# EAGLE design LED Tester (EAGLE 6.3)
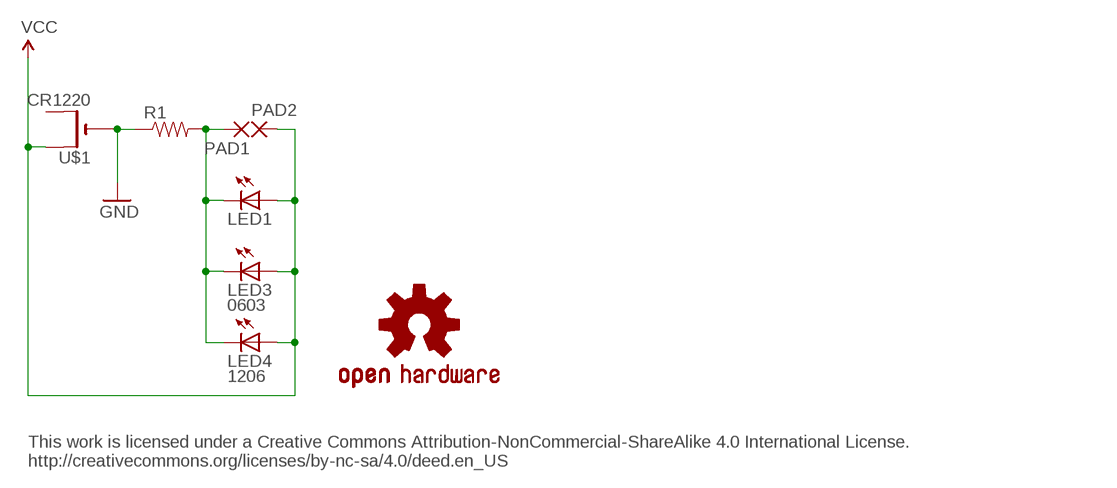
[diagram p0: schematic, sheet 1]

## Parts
LED1  LED3MM  [LED3MM]
LED3  0603  LED0603  [LED-0603]
LED4  1206  LED1206  [LED-1206]
LOGO1  OSHW-LOGOS  [OSHW-LOGO-S]
PAD1  SMD5  [SMD2,54-5,08]
PAD2  SMD5  [SMD2,54-5,08]
R1  RESISTOR0805-RES  [0805]
U$1  CR1220  CR1220THM  [CR1220-THM]

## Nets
GND: R1.1 U$1.-
N$1: LED1.K(C) LED3.C LED4.C PAD1.1(P) R1.2
VCC: LED1.A LED3.A LED4.A PAD2.1(P) U$1.+1(+)
Unconnected: U$1.+2(+1)

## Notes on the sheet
- This work is licensed under a Creative Commons Attribution-NonCommercial-ShareAlike 4.0 International License.
  http://creativecommons.org/licenses/by-nc-sa/4.0/deed.en_US

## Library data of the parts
LED1 LED3 LED4 = SparkFun-LED:LED: LEDs
LOGO1 = SparkFun-Aesthetics:OSHW-LOGO: Open Source Hardware Logo This logo indicates the piece of hardware it is found on incorporates a OSHW license and/or adheres to the definition of open source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
PAD1 PAD2 = wirepad:SMD5: SMD PAD
R1 = SparkFun-Resistors:RESISTOR: Resistor
U$1 = adafruit:CR1220: CR1216/CR1220/CR1225 12mm 3V lithium coin cell Great for battery packup. Both SMT and THM holders. Note the THM package has the ground pads on both sides of the PCB so that the masks are the same - this reduces the cost

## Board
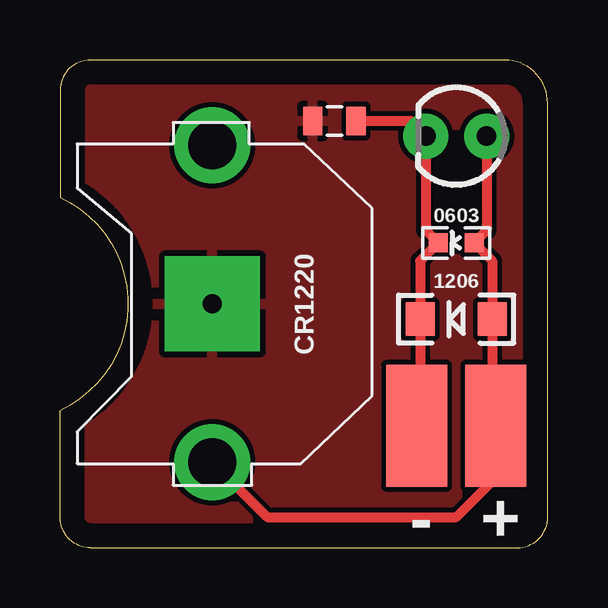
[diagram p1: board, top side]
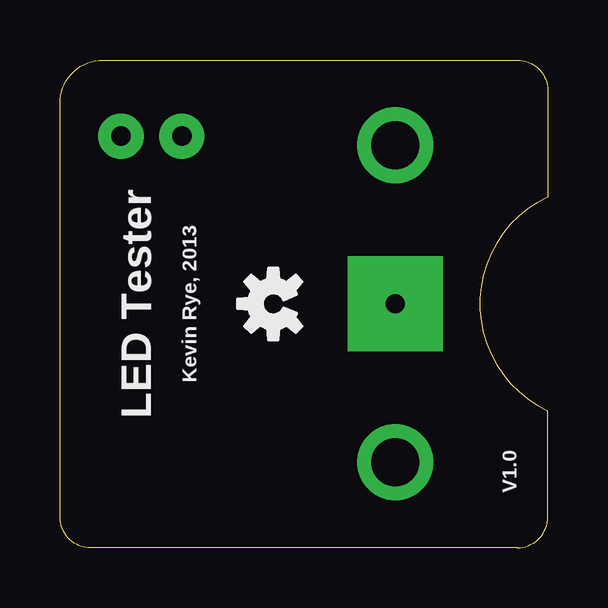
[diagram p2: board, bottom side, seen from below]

Size 20.32 x 20.32 mm. Coordinates in mm from the lower left corner, seen from the top.
Outline: 1.27,0 19.05,0 arc90 20.32,1.27 20.32,18.52 arc90 18.52,20.32 1.27,20.32 arc90 0,19.05 0,14.61 arc-130 0,5.71 0,1.27 arc90 1.27,0
Copper layers (1*16): Top 0.035mm / dielectric 1.5mm / Bottom 0.035mm
Design rules "default": minimum track width 10mil, minimum drill 24mil, track to track 8mil, track to pad 8mil, pad to pad 8mil, via to via 8mil, smd to smd 8mil, copper to edge 40mil, drill to drill 8mil, minimum pad ring 10mil, minimum via ring 8mil, stop-mask expansion 4mil, vias tented up to drill 0mil, thermal gap 10mil

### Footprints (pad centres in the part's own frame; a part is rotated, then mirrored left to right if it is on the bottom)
LED3MM = drill 0.813 pad 1.88: A -1.27,0; K 1.27,0
LED-0603 = smd 0.8 x 0.8: A 0,-0.75; C 0,0.75
LED-1206 = smd 1.2 x 1.4: A -1.5,0; C 1.5,0
SMD2,54-5,08 = smd 2.54 x 5.08: 1 0,0
0805 = smd 0.8 x 1.2: 1 -0.9,0; 2 0.9,0
CR1220-THM = drill 2 pad 3.175: +1 -6.604,0; +2 6.604,0 | drill 0.8 pad 3.962 square: - 0,0

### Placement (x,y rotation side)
LED1  16.51,17.14 180 top
LED3  16.51,12.7 90 top
LED4  16.51,9.53 180 top
LOGO1  11.43,10.16 90 bottom
PAD1  14.86,5.08 0 top
PAD2  18.16,5.08 0 top
R1  11.43,17.78 0 top
U$1  6.35,10.16 90 top

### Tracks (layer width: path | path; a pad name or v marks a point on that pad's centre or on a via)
GND
  pour Top: -2.54,22.86 22.86,22.86 22.86,-2.54 -2.54,-2.54
N$1
  Top 0.406: R1.2 14.61,17.78 LED1.K 15.24,13.22 LED3.C 15.01,11.95 LED4.C 15.01,6.35 15.24,6.35 15.24,5.08 PAD1.1
VCC
  Top 0.406: LED1.A 17.78,13.22 LED3.A 18.01,11.95 LED4.A 18.01,5.08 PAD2.1 18.16,2.92 16.51,1.27 8.64,1.27 U$1.+1

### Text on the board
Unrouted: This work is licensed under a Creative Commons Attribution-NonCommercial-ShareAlike 4.0 International License. / http://creativecommons.org/licenses/by-nc-sa/4.0/deed.en_US
tNames: - | +
bNames: Kevin Rye, 2013 | LED Tester | V1.0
